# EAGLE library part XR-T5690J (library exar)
T1/ISDN PRIMARY RATE FRAMER
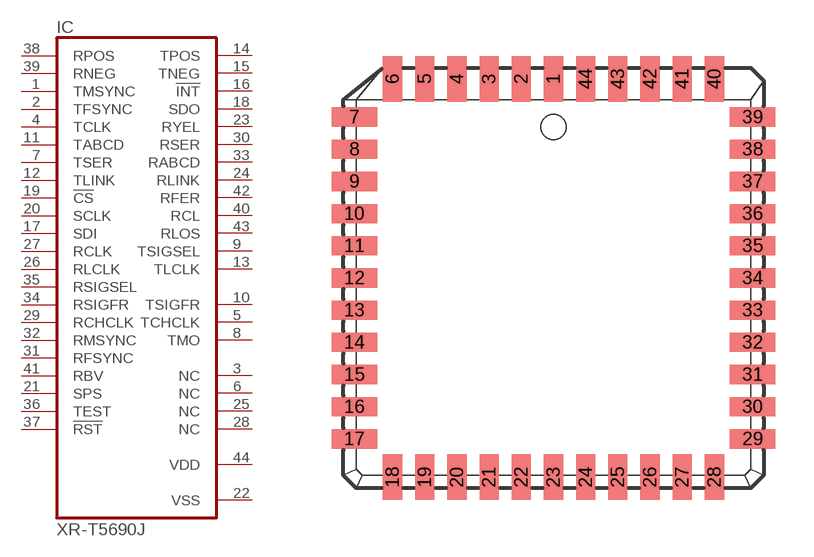
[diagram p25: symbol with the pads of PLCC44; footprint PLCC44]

Designator prefix IC

## XR-T5690J (OC_FARNELL: unknown; OC_NEWARK: unknown)  [PLCC44]
1  TMSYNC  in
2  TFSYNC  in
3  NC  nc
4  TCLK  in
5  TCHCLK  out
6  NC  nc
7  TSER  in
8  TMO  out
9  TSIGSEL  out
10  TSIGFR  out
11  TABCD  in
12  TLINK  in
13  TLCLK  out
14  TPOS  out
15  TNEG  out
16  !INT  out
17  SDI  in
18  SDO  out
19  !CS  in
20  SCLK  in
21  SPS  in
22  VSS  pwr
23  RYEL  out
24  RLINK  out
25  NC  nc
26  RLCLK  in
27  RCLK  in
28  NC  nc
29  RCHCLK  in
30  RSER  out
31  RFSYNC  in
32  RMSYNC  in
33  RABCD  out
34  RSIGFR  in
35  RSIGSEL  in
36  TEST  in
37  !RST  in
38  RPOS  in
39  RNEG  in
40  RCL  out
41  RBV  in
42  RFER  out
43  RLOS  out
44  VDD  pwr

## Footprint PLCC44 (pad centres in mm)
Plastic Leaded Chip Carrier
smd 0.76 x 1.8: 1 0,7.86; 2 -1.27,7.86; 3 -2.54,7.86; 4 -3.81,7.86; 5 -5.08,7.86; 6 -6.35,7.86; 18 -6.35,-7.86; 19 -5.08,-7.86; 20 -3.81,-7.86; 21 -2.54,-7.86; 22 -1.27,-7.86; 23 0,-7.86; 24 1.27,-7.86; 25 2.54,-7.86; 26 3.81,-7.86; 27 5.08,-7.86; 28 6.35,-7.86; 40 6.35,7.86; 41 5.08,7.86; 42 3.81,7.86; 43 2.54,7.86; 44 1.27,7.86
smd 1.8 x 0.76: 7 -7.86,6.35; 8 -7.86,5.08; 9 -7.86,3.81; 10 -7.86,2.54; 11 -7.86,1.27; 12 -7.86,0; 13 -7.86,-1.27; 14 -7.86,-2.54; 15 -7.86,-3.81; 16 -7.86,-5.08; 17 -7.86,-6.35; 29 7.86,-6.35; 30 7.86,-5.08; 31 7.86,-3.81; 32 7.86,-2.54; 33 7.86,-1.27; 34 7.86,0; 35 7.86,1.27; 36 7.86,2.54; 37 7.86,3.81; 38 7.86,5.08; 39 7.86,6.35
